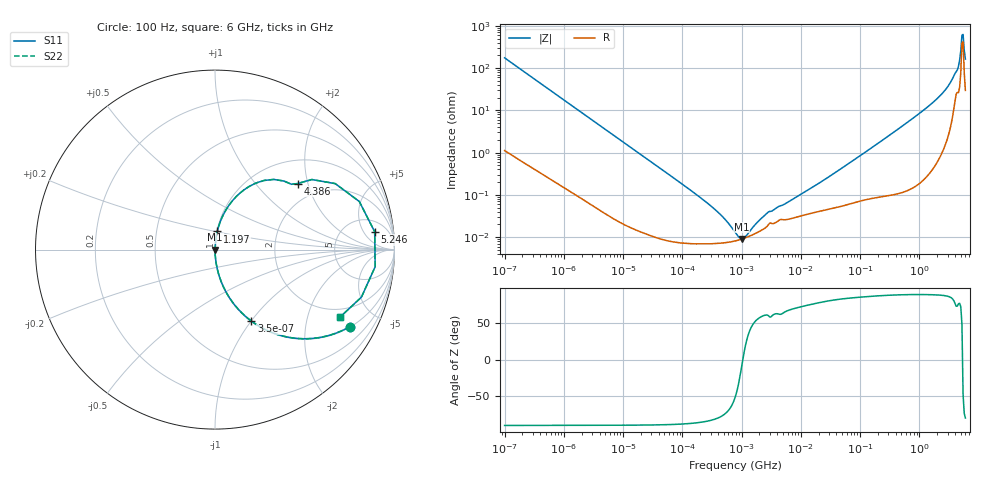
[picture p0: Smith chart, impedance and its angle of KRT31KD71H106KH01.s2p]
!Murata Part Number: KRT31KD71H106KH01
!These Parameters are Measured in Series Mode Connection
!Data Generated on Jan 08, 2026
!  o--ll--o
!Port1  Port2
!  o------o
!Operation Temp=25[degC], DC Bias Voltage=0[V]
!Freq. Start=100[Hz] Stop=6[GHz] 401[Steps]
# Hz S RI R 50
!Freq.(Hz) S11(Real) S11(Imag) S21(Real) S21(Imag) S12(Real) S12(Imag) S22(Real) S22(Imag)
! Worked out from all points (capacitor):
!   401 points, 100 Hz to 6 GHz, reference 50 ohm
!   read as one part in series: C = 9.09 uF near 109 Hz
!   lowest |Z| = 9.09 mohm at 1.013 MHz (marker M1)
!   series resonance near 1.049 MHz, so ESL is about 2.5 nH
!   S11 on the Smith chart (normalised r, x): 100 Hz: 1.02, -3.49; 350 Hz: 1.01, -1.00; 1.197 GHz: 1.00, +0.20; 4.386 GHz: 1.53, +1.72; 5.246 GHz: 9, +9; 6 GHz: 1.59, -3.21
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100  0.7518 -0.4288  0.2482 0.4288  0.2482 0.4288  0.7518 -0.4288
187  0.4671 -0.4955  0.5329 0.4955  0.5329 0.4955  0.4671 -0.4955
350  0.2027 -0.3983  0.7973 0.3983  0.7973 0.3983  0.2027 -0.3983
717  0.0586 -0.2309  0.9414 0.2309  0.9414 0.2309  0.0586 -0.2309
2008  0.00852 -0.0874  0.9915 0.0874  0.9915 0.0874  0.00852 -0.0874
40335  0.000113 -0.00446  0.9999 0.00446  0.9999 0.00446  0.000113 -0.00446
316350  7.03e-05 -0.000517  0.9999 0.000517  0.9999 0.000517  7.03e-05 -0.000517
517687  7.38e-05 -0.000261  0.9999 0.000261  0.9999 0.000261  7.38e-05 -0.000261
774597  8.13e-05 -0.000103  0.9999 0.000103  0.9999 0.000103  8.13e-05 -0.000103
1013323  9.02e-05 -1.15e-05  0.9999 1.15e-05  0.9999 1.15e-05  9.02e-05 -1.15e-05
1212075  9.88e-05 4.72e-05  0.9999 -4.72e-05  0.9999 -4.72e-05  9.88e-05 4.72e-05
2713602  0.000182 0.000326  0.9998 -0.000326  0.9998 -0.000326  0.000182 0.000326
1.555665e7  0.000374 0.00145  0.9996 -0.00145  0.9996 -0.00145  0.000374 0.00145
3.124326e8  0.00162 0.0256  0.9984 -0.0256  0.9984 -0.0256  0.00162 0.0256
1.197065e9  0.0126 0.101  0.9874 -0.101  0.9874 -0.101  0.0126 0.101
2.802721e9  0.1024 0.2782  0.8976 -0.2782  0.8976 -0.2782  0.1024 0.2782
3.505958e9  0.2286 0.3709  0.7714 -0.3709  0.7714 -0.3709  0.2286 0.3709
4.385646e9  0.4603 0.3681  0.5397 -0.3681  0.5397 -0.3681  0.4603 0.3681
4.796499e9  0.6702 0.3676  0.3298 -0.3676  0.3298 -0.3676  0.6702 0.3676
5.245841e9  0.8896 0.0997  0.1104 -0.0997  0.1104 -0.0997  0.8896 0.0997
5.737278e9  0.8159 -0.2647  0.1841 0.2647  0.1841 0.2647  0.8159 -0.2647
6e9  0.696 -0.3768  0.304 0.3768  0.304 0.3768  0.696 -0.3768
